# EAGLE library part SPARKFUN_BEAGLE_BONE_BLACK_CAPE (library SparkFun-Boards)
BeagleBone Black Rev C Cape Generic footprint for BeagleBone Black Rev C Capes. SparkFun Products: SparkFun BeagleBone Black Proto Cape SparkFun CryptoCape
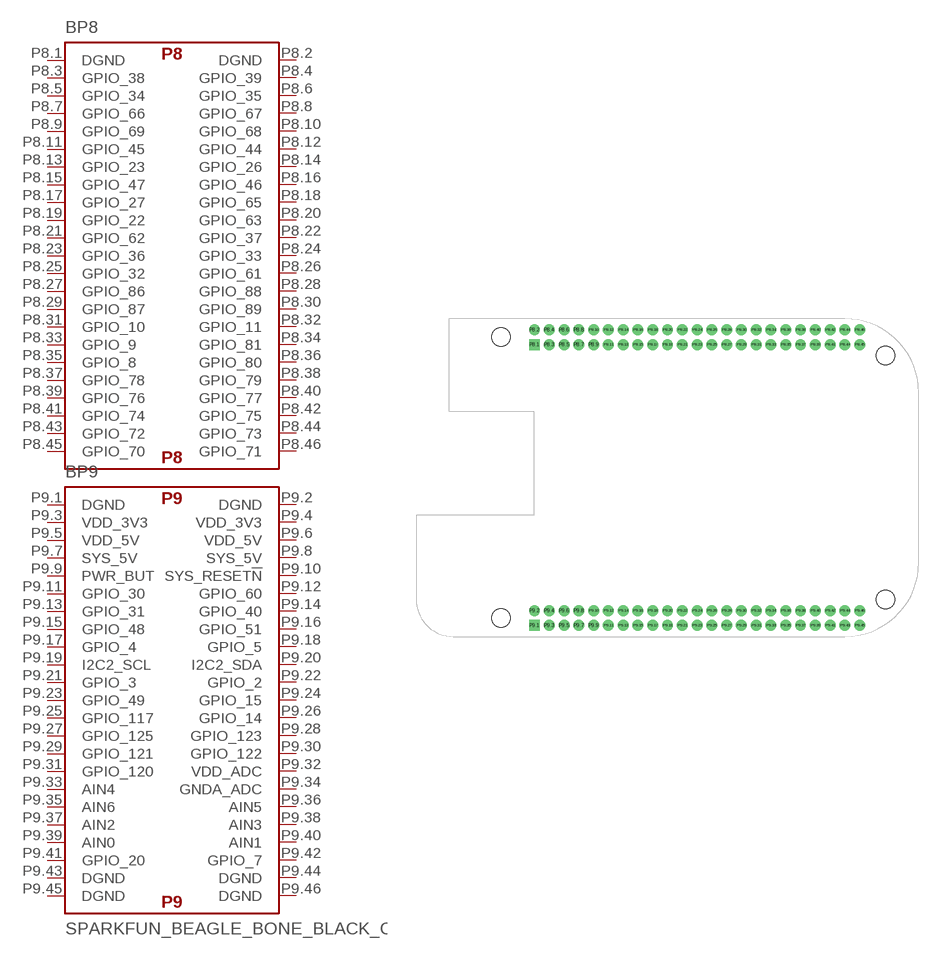
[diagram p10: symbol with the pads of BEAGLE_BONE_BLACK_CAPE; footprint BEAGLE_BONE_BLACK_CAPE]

Designator prefix B; gates P8=BEAGLE_BONE_BLACK_P8 P9=BEAGLE_BONE_BLACK_P9

## SPARKFUN_BEAGLE_BONE_BLACK_CAPE  [BEAGLE_BONE_BLACK_CAPE]
P8.1  P8:DGND
P8.2  P8:DGND
P8.3  P8:GPIO_38
P8.4  P8:GPIO_39
P8.5  P8:GPIO_34
P8.6  P8:GPIO_35
P8.7  P8:GPIO_66
P8.8  P8:GPIO_67
P8.9  P8:GPIO_69
P8.10  P8:GPIO_68
P8.11  P8:GPIO_45
P8.12  P8:GPIO_44
P8.13  P8:GPIO_23
P8.14  P8:GPIO_26
P8.15  P8:GPIO_47
P8.16  P8:GPIO_46
P8.17  P8:GPIO_27
P8.18  P8:GPIO_65
P8.19  P8:GPIO_22
P8.20  P8:GPIO_63
P8.21  P8:GPIO_62
P8.22  P8:GPIO_37
P8.23  P8:GPIO_36
P8.24  P8:GPIO_33
P8.25  P8:GPIO_32
P8.26  P8:GPIO_61
P8.27  P8:GPIO_86
P8.28  P8:GPIO_88
P8.29  P8:GPIO_87
P8.30  P8:GPIO_89
P8.31  P8:GPIO_10
P8.32  P8:GPIO_11
P8.33  P8:GPIO_9
P8.34  P8:GPIO_81
P8.35  P8:GPIO_8
P8.36  P8:GPIO_80
P8.37  P8:GPIO_78
P8.38  P8:GPIO_79
P8.39  P8:GPIO_76
P8.40  P8:GPIO_77
P8.41  P8:GPIO_74
P8.42  P8:GPIO_75
P8.43  P8:GPIO_72
P8.44  P8:GPIO_73
P8.45  P8:GPIO_70
P8.46  P8:GPIO_71
P9.1  P9:DGND
P9.2  P9:DGND
P9.3  P9:VDD_3V3
P9.4  P9:VDD_3V3
P9.5  P9:VDD_5V
P9.6  P9:VDD_5V
P9.7  P9:SYS_5V
P9.8  P9:SYS_5V
P9.9  P9:PWR_BUT
P9.10  P9:SYS_RESET!N
P9.11  P9:GPIO_30
P9.12  P9:GPIO_60
P9.13  P9:GPIO_31
P9.14  P9:GPIO_40
P9.15  P9:GPIO_48
P9.16  P9:GPIO_51
P9.17  P9:GPIO_4
P9.18  P9:GPIO_5
P9.19  P9:I2C2_SCL
P9.20  P9:I2C2_SDA
P9.21  P9:GPIO_3
P9.22  P9:GPIO_2
P9.23  P9:GPIO_49
P9.24  P9:GPIO_15
P9.25  P9:GPIO_117
P9.26  P9:GPIO_14
P9.27  P9:GPIO_125
P9.28  P9:GPIO_123
P9.29  P9:GPIO_121
P9.30  P9:GPIO_122
P9.31  P9:GPIO_120
P9.32  P9:VDD_ADC
P9.33  P9:AIN4
P9.34  P9:GNDA_ADC
P9.35  P9:AIN6
P9.36  P9:AIN5
P9.37  P9:AIN2
P9.38  P9:AIN3
P9.39  P9:AIN0
P9.40  P9:AIN1
P9.41  P9:GPIO_20
P9.42  P9:GPIO_7
P9.43  P9:DGND
P9.44  P9:DGND
P9.45  P9:DGND
P9.46  P9:DGND

## Footprint BEAGLE_BONE_BLACK_CAPE (pad centres in mm)
BeagleBone Black Cape Footprint Specifications: Pin count:92 Pin pitch: 0.1" Area:3.4x2.15 in Datasheet referenced for footprint: Example device(s): BeagleBone Black Cape
drill 1.016 pad 1.88 square: P8.1 -24.13,20.955; P9.1 -24.13,-27.305
drill 1.016 pad 1.88: P8.2 -24.13,23.495; P8.3 -21.59,20.955; P8.4 -21.59,23.495; P8.5 -19.05,20.955; P8.6 -19.05,23.495; P8.7 -16.51,20.955; P8.8 -16.51,23.495; P8.9 -13.97,20.955; P8.10 -13.97,23.495; P8.11 -11.43,20.955; P8.12 -11.43,23.495; P8.13 -8.89,20.955; P8.14 -8.89,23.495; P8.15 -6.35,20.955; P8.16 -6.35,23.495; P8.17 -3.81,20.955; P8.18 -3.81,23.495; P8.19 -1.27,20.955; P8.20 -1.27,23.495; P8.21 1.27,20.955; P8.22 1.27,23.495; P8.23 3.81,20.955; P8.24 3.81,23.495; P8.25 6.35,20.955; P8.26 6.35,23.495; P8.27 8.89,20.955; P8.28 8.89,23.495; P8.29 11.43,20.955; P8.30 11.43,23.495; P8.31 13.97,20.955; P8.32 13.97,23.495; P8.33 16.51,20.955; P8.34 16.51,23.495; P8.35 19.05,20.955; P8.36 19.05,23.495; P8.37 21.59,20.955; P8.38 21.59,23.495; P8.39 24.13,20.955; P8.40 24.13,23.495; P8.41 26.67,20.955; P8.42 26.67,23.495; P8.43 29.21,20.955; P8.44 29.21,23.495; P8.45 31.75,20.955; P8.46 31.75,23.495; P9.2 -24.13,-24.765; P9.3 -21.59,-27.305; P9.4 -21.59,-24.765; P9.5 -19.05,-27.305; P9.6 -19.05,-24.765; P9.7 -16.51,-27.305; P9.8 -16.51,-24.765; P9.9 -13.97,-27.305; P9.10 -13.97,-24.765; P9.11 -11.43,-27.305; P9.12 -11.43,-24.765; P9.13 -8.89,-27.305; P9.14 -8.89,-24.765; P9.15 -6.35,-27.305; P9.16 -6.35,-24.765; P9.17 -3.81,-27.305; P9.18 -3.81,-24.765; P9.19 -1.27,-27.305; P9.20 -1.27,-24.765; P9.21 1.27,-27.305; P9.22 1.27,-24.765; P9.23 3.81,-27.305; P9.24 3.81,-24.765; P9.25 6.35,-27.305; P9.26 6.35,-24.765; P9.27 8.89,-27.305; P9.28 8.89,-24.765; P9.29 11.43,-27.305; P9.30 11.43,-24.765; P9.31 13.97,-27.305; P9.32 13.97,-24.765; P9.33 16.51,-27.305; P9.34 16.51,-24.765; P9.35 19.05,-27.305; P9.36 19.05,-24.765; P9.37 21.59,-27.305; P9.38 21.59,-24.765; P9.39 24.13,-27.305; P9.40 24.13,-24.765; P9.41 26.67,-27.305; P9.42 26.67,-24.765; P9.43 29.21,-27.305; P9.44 29.21,-24.765; P9.45 31.75,-27.305; P9.46 31.75,-24.765
hole 3.175 at -29.845,-26.035
hole 3.175 at 36.195,-22.86
hole 3.175 at 36.195,19.05
hole 3.175 at -29.845,22.225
